//FB741.AWL
// ***************************************************************************

FUNCTION_BLOCK "ASTA_START_FB"
TITLE = Ablaufkettenstart

AUTHOR: 	SIEMENS
FAMILY: 	SISTARS7
NAME :    ASTA_FC
VERSION: 	4.02

//KNOW_HOW_PROTECT

//Historie:
//
// Datum     Name	Tätigkeit
//----------------------------------------------------------------------------
// 31.10.97  Vetter	Neu
// 04.11.97	 Vetter	Auswertung Fehler bei Remote Start
// 28.06.99	 Mahler	Ebene 4 Schnittstelle

VAR

	iType			:	INT	:= 1;		//DB-Type
	iOffset		:	INT	:= 300;	//Start 1. Datensatz
	iLen			:	INT	:= 20;	//Datensatzlänge
	iMax			:	INT	:= 96;	//max. Anzahl Datensätze
	iAct			:	INT	:= 96;	//aktuelle Anzahl Datensätze
	iRunOffset		:	INT	:= 100;	//Offset Bearbeitungsdatensatz
	iRecord		:	INT;			//1..n Nummer des aktuellen Datensatzes
	iStart		:	INT;
	abyFille		:	ARRAY  [1 .. 84 ] OF BYTE ;

	u			:	"ASTA_UDT";	//Bearbeitungsdatensatz

END_VAR


VAR_TEMP
	dwAR1			: DWORD;
	dSrcByte		: DINT;
	dDestByte		: DINT;
	i			: INT;
	iRetVal		: INT;
END_VAR

BEGIN

NETWORK
TITLE = Init.
// ===========================================================================

	TAR1	#dwAR1;


NETWORK
TITLE = Ziel-Teilanlage im eigenen AG
// ===========================================================================

	L	9;
	L	#u.bType;
	<=I;
	SPB	REM;

	L	0;
	L	#u.u.bDestSEQ;
	==I;
	SPB	ERR;
	T	#i;

	CALL	"ATTRIB_PTR_FC"
	(
  		iDB 			:= 725,
		iRecord 		:= i,
  		iRelByteOffset 	:= 0,
  		iRetVal 		:= #iRetVal
	);

	L	#iRetVal;
	L	0;
	<>I;
	SPB	ERR;

	AUF	"TA";

	UN	DBX	[AR1, P#7.6];		//TA: boDB Dauerbedingung nicht erfüllt
	SPB	ERR;

	U	DBX	[AR1, P#7.7];		//TA: boHAND Handbetrieb
	SPB	ERR;

	L	DBW	[AR1, P#10.0];		//TA: byNewStep, byStep
	L	0;
	<>I;
	SPB	ERR;					//Teilanlage läuft

	//Alles claro, TA kann gestartet werden
	l 0;
	T	#u.bRemoteError;
	T	#u.bRemoteOK;

	L	#u.u.bYear;
	T	DBB	[AR1, P#14.0];		//TA: byYear

	L	#u.u.bRecipeType;
	T	DBB	[AR1, P#15.0];		//TA: byRecType

	L	#u.u.iRecipe;
	T	DBW	[AR1, P#16.0];		//TA: iRecipe

	L	0;
	L	#u.u.iOrder;
	>=I;
	SPB	BAT;
	T	DBW	[AR1, P#18.0];		//TA: iOrder

BAT:	L	0;
	L	#u.u.iBatch;
	>=I;
	SPB	STEP;
	T	DBW	[AR1, P#20.0];		//TA: iBatch

STEP:	L	1;
	T	DBB	[AR1, P#10.0];		//TA: byNewStep

	SPA	OK;


NETWORK
TITLE = Ziel-Teilanlage im fremden AG
// ===========================================================================

REM:	NOP	0;

	L	"SYS".u.byAs;
	T	#u.u.bSrcPCU;

	L	#iRecord;
	T	#u.u.bSrcASTA;
	+	-1;
	L	#iLen;
	*I;
	L	#iOffset;
	+I;
	+	8;
	T	#dSrcByte;

	L	#u.u.bDestSEQ;
	+	-1;
	L	"XC_ASTA_RCV".iLen;
	*I;
	L	"XC_ASTA_RCV".iOffset;
	+I;
	T	#dDestByte;

	L	#u.u.bDestPCU;
	T	#i;

      u      #u.boSendRecv;			//Kennung Ebene 4 Schnittstelle
	spb 	E4;

	CALL	"XC_JOB_USER_IF_FC"		//Systemauftrag fuer Ebene 7
	(
		iMode			:= 1,
		iJob			:= 0,
		iPCU			:= #i,
		iType			:= 15,			//PUT
		boEnable		:= TRUE,
		boTmpJob		:= TRUE,
		iSrc_DType		:= 2,				//BYTE
		iSrc_AREA		:= 132,			//DB
		iSrc_DB		:= 742,			//"ASTA"
		dSrcByte		:= #dSrcByte,		//
		iSrcBit		:= 0,
		iSrc_Num		:= 12,
		iDest_DType		:= 2,				//BYTE
		iDest_AREA		:= 132,			//DB
		iDest_DB		:= 740,			//DB-Nummer
		dDestByte		:= #dDestByte,		//"XC_ASTA_RCV"
		iDestBit		:= 0,
		iTime			:= 0,
		iActTime		:= 0,
		iRetVal		:= #iRetVal
	);
	spa ret;

E4:	CALL	"FC_SR_JOB_USER"			//Systemauftrag fuer Ebene 4
	(
		iMode			:= 1,
		iJob			:= 0,
		iPCU			:= #i,
		iType			:= 54,			//Kettenstart
		boEnable		:= TRUE,
		boTmpJob		:= TRUE,
		iSrc_DType		:= 2,				//BYTE
		iSrc_AREA		:= 132,			//DB
		iSrc_DB		:= 742,			//"ASTA"
		dSrcByte		:= #dSrcByte,
		iSrcBit		:= 0,
		iSrc_Num		:= 12,
		iDest_DType		:= 2,				//BYTE
		iDest_AREA		:= 132,			//DB
		iDest_DB		:= 740,			//"XC_ASTA_RCV"
		dDestByte		:= #dDestByte,
		iDestBit		:= 0,
		iTime			:= 0,
		iActTime		:= 0,
		boTms			:= 0,
		boTsec		:= 0,
		boTmin		:= 0,
		iRetVal		:= #iRetVal
	);


ret:	L	#iRetVal;		//<=0: Fehler; >0: Belegter XC_JOB-Datensatz
	L	0;
	>I;
	SPB	OK;

NETWORK
TITLE = Fin de programma
// ===========================================================================

ERR:	SET;
	SPA	LAR;

OK:	CLR;

LAR:	LAR1	#dwAR1;


END_FUNCTION_BLOCK
